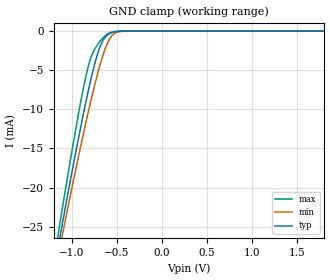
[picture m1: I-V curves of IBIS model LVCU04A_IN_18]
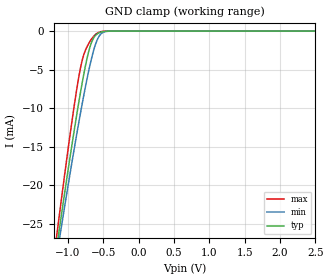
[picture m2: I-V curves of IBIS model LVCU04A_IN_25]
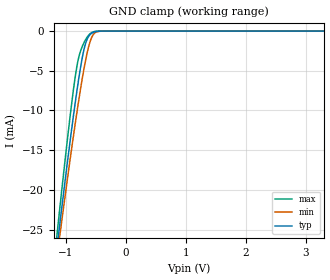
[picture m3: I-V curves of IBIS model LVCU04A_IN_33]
| TEXAS INSTRUMENTS INCORPORATED
| Standard Linear and Logic Group
| IBIS Model of SN74LVCU04A
| HEX INVERTER
| This file contains package information for the following:
|  SOIC 14-pin (D) package as [Component] LVCU04A_D
|  SSOP 14-pin (DB) package as [Component] LVCU04A_DB
|  TVSOP 14-pin (DGV) package as [Component] LVCU04A_DGV
|  SOP 14-pin (NS) package as [Component] LVCU04A_NS
|  TSSOP 14-pin (PW) package as [Component] LVCU04A_PW
| This device can be powered at the following Vccs:
|  1.8 volt Vcc
|  2.5 volt Vcc
|  3.3 volt Vcc
| This file provides unique models under the [Model Selector] for each Vcc.
| For operation at a specific Vcc, select the appropriate model after each
| [Model Selector] keyword.
[IBIS Ver]   3.2
[Comment char]  |_char
[File Name]   sn74lvcu04a.ibs
[File Rev]   1.1 | k_die
[Date]   April 29, 2002
[Source]   Data created from TI-SPICE simulations at TI-SLL.
[Notes]   The following is an IBIS list for the SN74LVCU04A.
   Please contact sllibis@ti.com with questions and
   comments concerning SLL IBIS models.
   - C_comp values are taken at a different test condition
   than the data sheet.
[Disclaimer] Property of Texas Instruments Incorporated.  Unauthorized
   reproduction and/or distribution is strictly prohibited.
   This product is protected under copyright law.
   Created  2002, (C) Copyright  2002, Texas Instruments
   Incorporated, All Rights Reserved
   UNLESS THERE IS A SIGNED, WRITTEN AGREEMENT TO THE
   CONTRARY, TEXAS INSTRUMENTS (TI) IS PROVIDING THE IBIS
   MODELS  AND WITHOUT ANY WARRANTY, EXPRESSED OR
   IMPLIED.  TI assumes no liability for:
   1) the accuracy of the IBIS models provided to your
   company;
   2) the proper functioning of these IBIS Models in your
   design or for any resulting applications; or
   3) infringement of patents, copyrights or intellectual
   property rights resulting from your use of these IBIS
   models.
   TI provides IBIS Models as a service to our customers.
   You and your company shall not distribute, sell or give
   these models to anyone else without prior written
   permission from TI.
   TI reserves the right to make changes to our products or
   to discontinue any semiconductor product or service
   without notice, and advises our customers to obtain the
   latest version of relevant information to verify, before
   placing orders, that the information being relied on is
   current.
   Please be aware that your receipt and use of the IBIS
   information provided shall serve as acceptance of these
   terms and conditions.  If you do not accept these terms,
   you should return or destroy the IBIS models and any
   other accompanying information immediately.
| Component LVCU04A_D 14-pin SOIC
[Component]   LVCU04A_D
[Manufacturer]  Texas Instruments, Inc.
[Package]
|   typ   min   max
R_pkg   3.100e-02   2.800e-02   3.400e-02
L_pkg   3.109e-09   2.462e-09   3.889e-09
C_pkg   4.730e-13   3.630e-13   6.280e-13
[Pin]   signal_name   model_name   R_pin   L_pin   C_pin
1   1A   LVCU04A_IN   3.300e-02   3.854e-09   6.220e-13
2   1Y   LVCU04A_OUT   3.200e-02   3.188e-09   4.730e-13
3   2A   LVCU04A_IN   2.800e-02   2.462e-09   3.770e-13
4   2Y   LVCU04A_OUT   3.100e-02   2.596e-09   3.630e-13
5   3A   LVCU04A_IN   2.800e-02   2.521e-09   3.720e-13
6   3Y   LVCU04A_OUT   3.400e-02   3.250e-09   4.760e-13
7   GND   GND   3.400e-02   3.889e-09   6.280e-13
8   4Y   LVCU04A_OUT   3.400e-02   3.889e-09   6.280e-13
9   4A   LVCU04A_IN   3.400e-02   3.250e-09   4.760e-13
10   5Y   LVCU04A_OUT   2.800e-02   2.521e-09   3.720e-13
11   5A   LVCU04A_IN   3.100e-02   2.596e-09   3.640e-13
12   6Y   LVCU04A_OUT   2.800e-02   2.462e-09   3.770e-13
13   6A   LVCU04A_IN   3.200e-02   3.188e-09   4.730e-13
14   VCC   POWER   3.300e-02   3.854e-09   6.220e-13
| Component LVCU04A_DB 14-pin SSOP
[Component]   LVCU04A_DB
[Manufacturer]  Texas Instruments, Inc.
[Package]
|   typ   min   max
R_pkg   4.400e-02   4.100e-02   4.600e-02
L_pkg   3.551e-09   3.258e-09   3.927e-09
C_pkg   4.020e-13   3.600e-13   4.210e-13
[Pin]   signal_name   model_name   R_pin   L_pin   C_pin
1   1A   LVCU04A_IN   4.600e-02   3.927e-09   4.080e-13
2   1Y   LVCU04A_OUT   4.400e-02   3.587e-09   4.210e-13
3   2A   LVCU04A_IN   4.100e-02   3.289e-09   3.980e-13
4   2Y   LVCU04A_OUT   4.200e-02   3.258e-09   3.600e-13
5   3A   LVCU04A_IN   4.100e-02   3.286e-09   4.030e-13
6   3Y   LVCU04A_OUT   4.400e-02   3.586e-09   4.210e-13
7   GND   GND   4.600e-02   3.927e-09   4.080e-13
8   4Y   LVCU04A_OUT   4.600e-02   3.927e-09   4.080e-13
9   4A   LVCU04A_IN   4.400e-02   3.586e-09   4.210e-13
10   5Y   LVCU04A_OUT   4.100e-02   3.286e-09   4.030e-13
11   5A   LVCU04A_IN   4.300e-02   3.258e-09   3.600e-13
12   6Y   LVCU04A_OUT   4.100e-02   3.289e-09   3.980e-13
13   6A   LVCU04A_IN   4.400e-02   3.587e-09   4.210e-13
14   VCC   POWER   4.600e-02   3.927e-09   4.080e-13
| Component LVCU04A_DGV 14-pin TVSOP
[Component]   LVCU04A_DGV
[Manufacturer]  Texas Instruments, Inc.
[Package]
|   typ   min   max
R_pkg   3.500e-02   2.000e-02   4.500e-02
L_pkg   2.499e-09   2.077e-09   2.966e-09
C_pkg   3.610e-13   3.050e-13   4.160e-13
[Pin]   signal_name   model_name   R_pin   L_pin   C_pin
1   1A   LVCU04A_IN   2.700e-02   2.717e-09   3.730e-13
2   1Y   LVCU04A_OUT   3.700e-02   2.434e-09   3.980e-13
3   2A   LVCU04A_IN   3.400e-02   2.200e-09   3.160e-13
4   2Y   LVCU04A_OUT   2.000e-02   2.077e-09   3.090e-13
5   3A   LVCU04A_IN   3.000e-02   2.147e-09   3.050e-13
6   3Y   LVCU04A_OUT   4.200e-02   2.580e-09   4.080e-13
7   GND   GND   3.900e-02   2.921e-09   3.850e-13
8   4Y   LVCU04A_OUT   3.300e-02   2.841e-09   3.800e-13
9   4A   LVCU04A_IN   4.200e-02   2.611e-09   4.100e-13
10   5Y   LVCU04A_OUT   3.800e-02   2.331e-09   3.290e-13
11   5A   LVCU04A_IN   2.600e-02   2.223e-09   3.190e-13
12   6Y   LVCU04A_OUT   3.400e-02   2.259e-09   3.130e-13
13   6A   LVCU04A_IN   4.500e-02   2.681e-09   4.160e-13
14   VCC   POWER   4.200e-02   2.966e-09   3.860e-13
| Component LVCU04A_NS 14-pin SOP
[Component]   LVCU04A_NS
[Manufacturer]  Texas Instruments, Inc.
[Package]
|   typ   min   max
R_pkg   4.500e-02   3.900e-02   5.400e-02
L_pkg   3.796e-09   2.561e-09   4.952e-09
C_pkg   5.280e-13   2.880e-13   7.100e-13
[Pin]   signal_name   model_name   R_pin   L_pin   C_pin
1   1A   LVCU04A_IN   4.700e-02   4.867e-09   7.060e-13
2   1Y   LVCU04A_OUT   5.100e-02   4.083e-09   5.920e-13
3   2A   LVCU04A_IN   4.100e-02   2.915e-09   3.760e-13
4   2Y   LVCU04A_OUT   3.900e-02   2.561e-09   2.880e-13
5   3A   LVCU04A_IN   4.100e-02   3.101e-09   4.300e-13
6   3Y   LVCU04A_OUT   4.700e-02   4.047e-09   5.890e-13
7   GND   GND   5.100e-02   4.909e-09   7.000e-13
8   4Y   LVCU04A_OUT   4.500e-02   4.784e-09   6.940e-13
9   4A   LVCU04A_IN   5.400e-02   4.176e-09   5.970e-13
10   5Y   LVCU04A_OUT   3.900e-02   3.287e-09   4.490e-13
11   5A   LVCU04A_IN   3.900e-02   2.586e-09   2.940e-13
12   6Y   LVCU04A_OUT   4.000e-02   2.802e-09   3.710e-13
13   6A   LVCU04A_IN   4.900e-02   4.080e-09   5.930e-13
14   VCC   POWER   5.200e-02   4.952e-09   7.100e-13
| Component LVCU04A_PW 14-pin TSSOP
[Component]   LVCU04A_PW
[Manufacturer]  Texas Instruments, Inc.
[Package]
|   typ   min   max
R_pkg   3.200e-02   2.900e-02   3.500e-02
L_pkg   2.378e-09   2.170e-09   2.680e-09
C_pkg   3.140e-13   2.700e-13   3.350e-13
[Pin]   signal_name   model_name   R_pin   L_pin   C_pin
1   1A   LVCU04A_IN   3.300e-02   2.618e-09   3.300e-13
2   1Y   LVCU04A_OUT   3.100e-02   2.313e-09   3.170e-13
3   2A   LVCU04A_IN   3.000e-02   2.310e-09   3.140e-13
4   2Y   LVCU04A_OUT   3.100e-02   2.173e-09   2.720e-13
5   3A   LVCU04A_IN   3.000e-02   2.204e-09   3.090e-13
6   3Y   LVCU04A_OUT   3.200e-02   2.315e-09   3.170e-13
7   GND   GND   3.500e-02   2.680e-09   3.350e-13
8   4Y   LVCU04A_OUT   3.300e-02   2.640e-09   3.330e-13
9   4A   LVCU04A_IN   3.400e-02   2.347e-09   3.190e-13
10   5Y   LVCU04A_OUT   2.900e-02   2.277e-09   3.130e-13
11   5A   LVCU04A_IN   3.100e-02   2.170e-09   2.700e-13
12   6Y   LVCU04A_OUT   3.100e-02   2.244e-09   3.110e-13
13   6A   LVCU04A_IN   3.300e-02   2.343e-09   3.210e-13
14   VCC   POWER   3.500e-02   2.657e-09   3.320e-13
| Model LVCU04A_IN
[Model Selector]   LVCU04A_IN
LVCU04A_IN_18   1.8 volt Vcc
LVCU04A_IN_25   2.5 volt Vcc
LVCU04A_IN_33   3.3 volt Vcc
| Model LVCU04A_OUT
[Model Selector]   LVCU04A_OUT
LVCU04A_OUT_18   1.8 volt Vcc
LVCU04A_OUT_25   2.5 volt Vcc
LVCU04A_OUT_33   3.3 volt Vcc
| Models and submodels in the file (6): LVCU04A_IN_18 (Input), LVCU04A_IN_25 (Input), LVCU04A_IN_33 (Input), LVCU04A_OUT_18 (Output), LVCU04A_OUT_25 (Output), LVCU04A_OUT_33 (Output)
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[Model]   LVCU04A_IN_18
Model_type  Input
Vinl=0.4
Vinh=1.32
| variable   typ   min   max
C_comp   2.63pF   2.15pF   3.12pF
[Temperature Range]   40   100   -40
| Ambient temperature   25   85   -40
[Voltage range]   1.8   1.65   1.95
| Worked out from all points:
|   GND clamp passes 1 mA (typ) near -0.64 V on its own axis
[GND Clamp]
| LVCU04A_IN_18
|   Voltage   I(typ)   I(min)   I(max)
-5.5V     -338.9mA   -314.3mA   -369mA
-1.16V    -28.09mA   -29.24mA   -26.56mA
-1.12V    -25.56mA   -26.92mA   -23.71mA
-1.085V   -23.36mA   -24.91mA   -21.25mA
-925mV    -13.65mA   -15.98mA   -10.52mA
-820mV    -7.797mA   -10.48mA   -4.654mA
-770mV    -5.293mA   -8.026mA   -2.891mA
-695mV    -2.253mA   -4.666mA   -1.432mA
-600mV    -473.7uA   -1.449mA   -358.4uA
-535mV    -136.2uA   -379.8uA   -78.5uA
-445mV    -16.2uA    -36.49uA   -4.833uA
1.8V      41.95pA    147.4pA    23.47pA
[Model]   LVCU04A_IN_25
Model_type  Input
Vinl=0.5
Vinh=1.84
| variable   typ   min   max
C_comp   2.57pF   2.09pF   3.19pF
[Temperature Range]   40   100   -40
| Ambient temperature   25   85   -40
[Voltage range]   2.5   2.3   2.7
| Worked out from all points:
|   GND clamp passes 1 mA (typ) near -0.64 V on its own axis
[GND Clamp]
| LVCU04A_IN_25
|   Voltage   I(typ)   I(min)   I(max)
-5.5V     -338.9mA   -314.3mA   -369mA
-1.17V    -28.73mA   -29.82mA   -27.27mA
-1.13V    -26.19mA   -27.5mA    -24.42mA
-1.095V   -23.98mA   -25.48mA   -21.95mA
-925mV    -13.65mA   -15.98mA   -10.52mA
-825mV    -8.06mA    -10.74mA   -4.88mA
-775mV    -5.531mA   -8.266mA   -3.027mA
-700mV    -2.416mA   -4.874mA   -1.51mA
-590mV    -396.4uA   -1.217mA   -293.2uA
-515mV    -88.16uA   -231.8uA   -44.89uA
-395mV    -4.232uA   -9.445uA   -775nA
2.5V      57.25pA    176.8pA    32.61pA
[Model]   LVCU04A_IN_33
Model_type  Input
Vinl=0.65
Vinh=2.4
| variable   typ   min   max
C_comp   2.49pF   1.95pF   3.19pF
[Temperature Range]   40   100   -40
| Ambient temperature   25   85   -40
[Voltage range]   3.3   3   3.6
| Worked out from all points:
|   GND clamp passes 1 mA (typ) near -0.64 V on its own axis
[GND Clamp]
| LVCU04A_IN_33
|   Voltage   I(typ)   I(min)   I(max)
-5.5V     -338.9mA   -314.3mA   -369mA
-1.14V    -26.82mA   -28.07mA   -25.13mA
-1.105V   -24.61mA   -26.05mA   -22.65mA
-1.075V   -22.73mA   -24.34mA   -20.55mA
-915mV    -13.07mA   -15.45mA   -9.893mA
-860mV    -9.954mA   -12.53mA   -6.658mA
-805mV    -7.019mA   -9.733mA   -4.027mA
-730mV    -3.528mA   -6.174mA   -2.02mA
-665mV    -1.428mA   -3.486mA   -1.009mA
-585mV    -362.1uA   -1.111mA   -263.9uA
-510mV    -78.77uA   -204.1uA   -38.82uA
3.3V      76.2pA     212.8pA    43.07pA
